(* Logix 5000 AddOnInstructionDefinition export Banner_K50ProTouch_PD_v4; software revision 33.00 *)

TYPE Banner_K50Pro_4State_v4 :   // Process Data for Four State Mode. This mode is only available in Touch models.
STRUCT
   Touch_Status : SINT;   // 0 = Inactive, 1 = Active. Only active for Touch models.
   In_State : SINT;   // Curent State. 0 = State 1, 1 = State 2, 2 = State 3, 3 = State 4
   Job_Control : SINT;   // 0 = Off, 1 = On
END_STRUCT
END_TYPE

TYPE Banner_K50Pro_MC_v4 :   // Process Data for Multicolor
STRUCT
   Touch_Status : SINT;   // 0 = Inactive, 1 = Active. Only active for Touch models.
   In_State : SINT;   // Curent State. 0 = State 1, 1 = State 2, 2 = State 3, 3 = State 4
   Out_State : SINT;   // Set Output State. 0 = State 1, 1 = State 2, 2 = State 3, 3 = State 4
END_STRUCT
END_TYPE

TYPE Banner_K50ProTouch_Adv_v4 :   // Advanced Process Data information for a Banner K50 Pro Touch.
STRUCT
   Touch_Status : SINT;   // 0 = Inactive, 1 = Active.
   Type : SINT;   // 0 = Off, 1 = Steady, 2 = Flash, 3 = Two Color Flash, 4 = 50/50, 5 = 50/50 Rotate, 6 = Chase, 7 = Intensity Sweep, 8 = Sequence.
   Direction : SINT;   // 0 = CCW, 1 = CW.
   Pattern : SINT;   // 0 = Flash, 1 = Strobe, 2 = Three Pulse, 3 = SOS, 4 = Random.
   Speed : SINT;   // 0 = Slow, 1 = Medium, 2 = Fast, 3 = Custom.
   Vibration_Feedback : SINT;   // 0 = Off, 1 = On, 2 = Animation Pattern. Not available in all models.
   Dynamic_Sequence : INT;   // 0 to 255. Value describing the LED position on the device.
   Sequence_Start_Location : SINT;   // 0 = LED 1, 1 = LED 2, 2 = LED 3, 3 = LED 4, 4 = LED 5, 5 = LED 6, 6 = LED 7, 7 = LED 8.
   Color_1 : SINT;   // 0 = Green, 1 = Red, 2 = Orange, 3 = Amber, 4 = Yellow, 5 = Lime Green, 6 = Spring Green, 7 = Cyan, 8 = Sky Blue, 9 = Blue, 10 = Violet, 11 = Magenta, 12 = Rose, 13 = White, 14 = Custom 1, 15 = Custom 2.
   Color_1_Intensity : SINT;   // 0 = High, 1 = Medium, 2 = Low, 3 = Off, 4 = Custom.
   Color_2 : SINT;   // 0 = Green, 1 = Red, 2 = Orange, 3 = Amber, 4 = Yellow, 5 = Lime Green, 6 = Spring Green, 7 = Cyan, 8 = Sky Blue, 9 = Blue, 10 = Violet, 11 = Magenta, 12 = Rose, 13 = White, 14 = Custom 1, 15 = Custom 2.
   Color_2_Intensity : SINT;   // 0 = High, 1 = Medium, 2 = Low, 3 = Off, 4 = Custom.
END_STRUCT
END_TYPE

TYPE Banner_K50ProTouch_LEDControl_v4 :   // LED Control Process Data for a K50 Pro Touch.
STRUCT
   Touch_Status : SINT;   // 0 = Inactive, 1 = Active.
   LED_1_Color : SINT;   // 0 = Green, 1 = Red, 2 = Orange, 3 = Amber, 4 = Yellow, 5 = Lime Green, 6 = Spring Green, 7 = Cyan, 8 = Sky Blue, 9 = Blue, 10 = Violet, 11 = Magenta, 12 = Rose, 13 = White, 14 = Custom 1, 15 = Custom 2.
   LED_1_Intensity : SINT;   // 0 to 10 (0 to 100%).
   LED_2_Color : SINT;   // 0 = Green, 1 = Red, 2 = Orange, 3 = Amber, 4 = Yellow, 5 = Lime Green, 6 = Spring Green, 7 = Cyan, 8 = Sky Blue, 9 = Blue, 10 = Violet, 11 = Magenta, 12 = Rose, 13 = White, 14 = Custom 1, 15 = Custom 2.
   LED_2_Intensity : SINT;   // 0 to 10 (0 to 100%).
   LED_3_Color : SINT;   // 0 = Green, 1 = Red, 2 = Orange, 3 = Amber, 4 = Yellow, 5 = Lime Green, 6 = Spring Green, 7 = Cyan, 8 = Sky Blue, 9 = Blue, 10 = Violet, 11 = Magenta, 12 = Rose, 13 = White, 14 = Custom 1, 15 = Custom 2.
   LED_3_Intensity : SINT;   // 0 to 10 (0 to 100%).
   LED_4_Color : SINT;   // 0 = Green, 1 = Red, 2 = Orange, 3 = Amber, 4 = Yellow, 5 = Lime Green, 6 = Spring Green, 7 = Cyan, 8 = Sky Blue, 9 = Blue, 10 = Violet, 11 = Magenta, 12 = Rose, 13 = White, 14 = Custom 1, 15 = Custom 2.
   LED_4_Intensity : SINT;   // 0 to 10 (0 to 100%).
   LED_5_Color : SINT;   // 0 = Green, 1 = Red, 2 = Orange, 3 = Amber, 4 = Yellow, 5 = Lime Green, 6 = Spring Green, 7 = Cyan, 8 = Sky Blue, 9 = Blue, 10 = Violet, 11 = Magenta, 12 = Rose, 13 = White, 14 = Custom 1, 15 = Custom 2.
   LED_5_Intensity : SINT;   // 0 to 10 (0 to 100%).
   LED_6_Color : SINT;   // 0 = Green, 1 = Red, 2 = Orange, 3 = Amber, 4 = Yellow, 5 = Lime Green, 6 = Spring Green, 7 = Cyan, 8 = Sky Blue, 9 = Blue, 10 = Violet, 11 = Magenta, 12 = Rose, 13 = White, 14 = Custom 1, 15 = Custom 2.
   LED_6_Intensity : SINT;   // 0 to 10 (0 to 100%).
   LED_7_Color : SINT;   // 0 = Green, 1 = Red, 2 = Orange, 3 = Amber, 4 = Yellow, 5 = Lime Green, 6 = Spring Green, 7 = Cyan, 8 = Sky Blue, 9 = Blue, 10 = Violet, 11 = Magenta, 12 = Rose, 13 = White, 14 = Custom 1, 15 = Custom 2.
   LED_7_Intensity : SINT;   // 0 to 10 (0 to 100%).
   LED_8_Color : SINT;   // 0 = Green, 1 = Red, 2 = Orange, 3 = Amber, 4 = Yellow, 5 = Lime Green, 6 = Spring Green, 7 = Cyan, 8 = Sky Blue, 9 = Blue, 10 = Violet, 11 = Magenta, 12 = Rose, 13 = White, 14 = Custom 1, 15 = Custom 2.
   LED_8_Intensity : SINT;   // 0 to 10 (0 to 100%).
   Vibration_Feedback : SINT;   // 0 = Off, 1 = On, 2 = Pattern.
   Vibration_Pattern : SINT;   // 0 = Off, 1 = On, 2 = 3 Pulses, 3 = SOS, 4 = Random.
   Vibration_Speed : SINT;   // 0 = Slow, 1 = Medium, 2 = Fast, 3 = Custom.
END_STRUCT
END_TYPE

TYPE Banner_K50ProTouch_PDIO_v4 :   // UDT that records the converted prcoess data.
STRUCT
   PD_MultiColor_State : Banner_K50Pro_MC_v4;   // Only active when Operation Mode set to 0. State tells the light which of the four states it should be in. 0 = State 1, 1 = State 2, 2 = State 3, 3 = State 4.
   PD_FourState_Job_Input : Banner_K50Pro_4State_v4;   // Only active when Operation Mode set to 1. Job Input tells the light how it should behave. 0 - Off, 1 = ON
   PD_Advanced : Banner_K50ProTouch_Adv_v4;   // Only active when Operation Mode set to 2.
   PD_LED : Banner_K50ProTouch_LEDControl_v4;   // Only active when Operation Mode set to 3.
   PDO_DT : SINT[10];
   PDI_DT : SINT[2];
END_STRUCT
END_TYPE

ADD_ON_INSTRUCTION Banner_K50ProTouch_PD_v4   (* revision 4.0, vendor Banner Engineering *)
// Takes the raw SINT information and converts that data into actual information.
VAR_IN_OUT
   Process_Data : Banner_K50ProTouch_PDIO_v4; {required}
END_VAR
VAR_INPUT
   Operation_Mode : SINT; {required}   // Linked from Parameters AOI or entered manually.
   Byte_Swap : BOOL; {required}
END_VAR
VAR
   PDO_Temp : SINT[10]; {access None}
   PDI_Temp : SINT[2]; {access None}
END_VAR

ROUTINE Logic   (* ladder *)
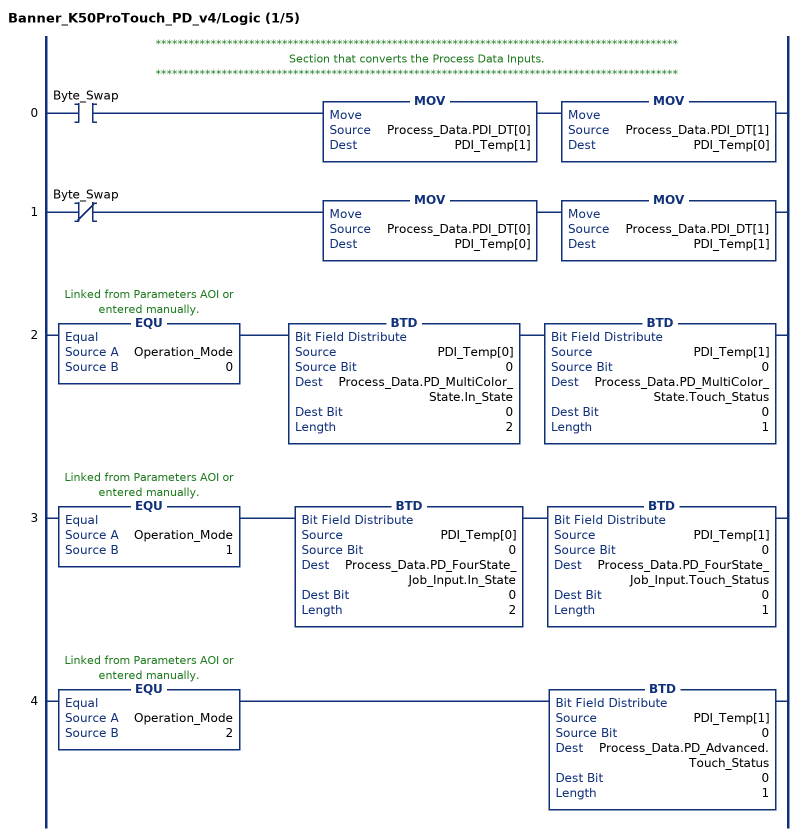
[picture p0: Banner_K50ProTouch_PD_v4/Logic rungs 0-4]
   // ***********************************************************************************************
   // Section that converts the Process Data Inputs.
   // ***********************************************************************************************
   0: XIC(Byte_Swap)MOV(Process_Data.PDI_DT[0],PDI_Temp[1])MOV(Process_Data.PDI_DT[1],PDI_Temp[0]);
   1: XIO(Byte_Swap)MOV(Process_Data.PDI_DT[0],PDI_Temp[0])MOV(Process_Data.PDI_DT[1],PDI_Temp[1]);
   2: EQU(Operation_Mode,0)BTD(PDI_Temp[0],0,Process_Data.PD_MultiColor_State.In_State,0,2)BTD(PDI_Temp[1],0,Process_Data.PD_MultiColor_State.Touch_Status,0,1);
   3: EQU(Operation_Mode,1)BTD(PDI_Temp[0],0,Process_Data.PD_FourState_Job_Input.In_State,0,2)BTD(PDI_Temp[1],0,Process_Data.PD_FourState_Job_Input.Touch_Status,0,1);
   4: EQU(Operation_Mode,2)BTD(PDI_Temp[1],0,Process_Data.PD_Advanced.Touch_Status,0,1);
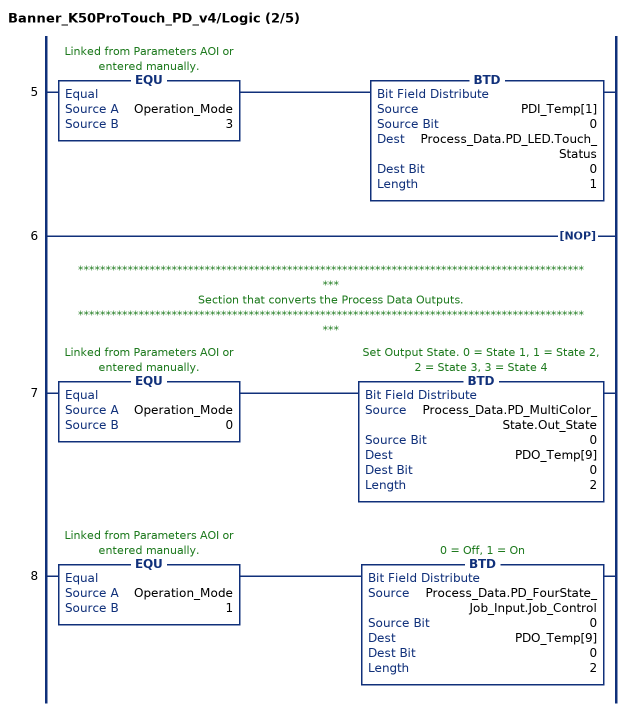
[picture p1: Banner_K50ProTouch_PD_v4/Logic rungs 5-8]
   5: EQU(Operation_Mode,3)BTD(PDI_Temp[1],0,Process_Data.PD_LED.Touch_Status,0,1);
   6: NOP();
   // ***********************************************************************************************
   // Section that converts the Process Data Outputs.
   // ***********************************************************************************************
   7: EQU(Operation_Mode,0)BTD(Process_Data.PD_MultiColor_State.Out_State,0,PDO_Temp[9],0,2);
   8: EQU(Operation_Mode,1)BTD(Process_Data.PD_FourState_Job_Input.Job_Control,0,PDO_Temp[9],0,2);
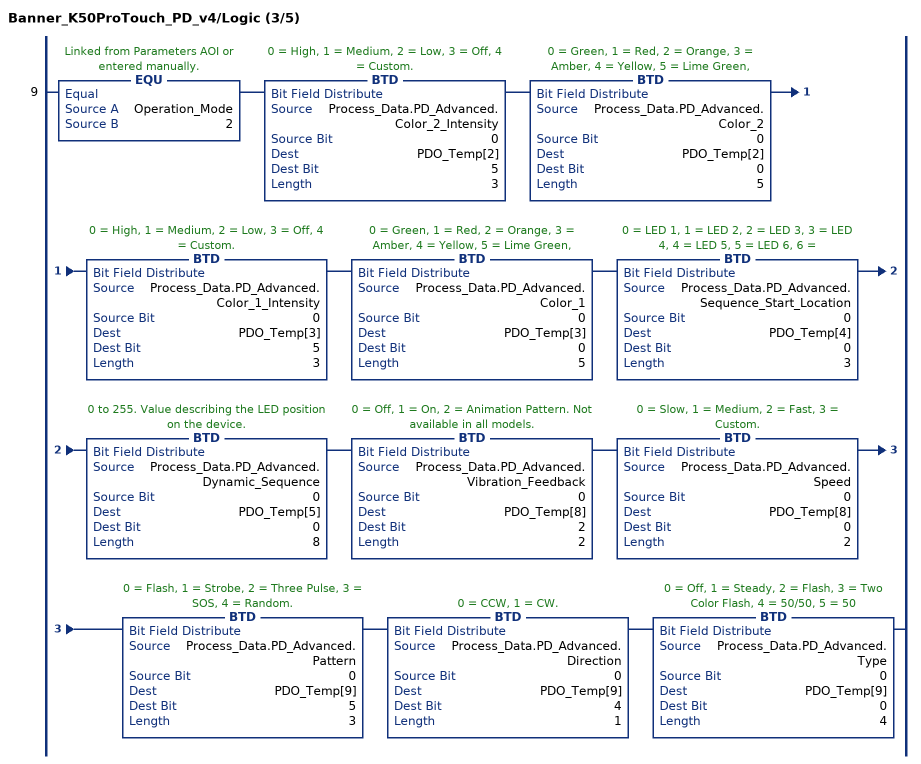
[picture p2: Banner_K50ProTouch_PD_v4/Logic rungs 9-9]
   9: EQU(Operation_Mode,2)BTD(Process_Data.PD_Advanced.Color_2_Intensity,0,PDO_Temp[2],5,3)BTD(Process_Data.PD_Advanced.Color_2,0,PDO_Temp[2],0,5)BTD(Process_Data.PD_Advanced.Color_1_Intensity,0,PDO_Temp[3],5,3)BTD(Process_Data.PD_Advanced.Color_1,0,PDO_Temp[3],0,5)BTD(Process_Data.PD_Advanced.Sequence_Start_Location,0,PDO_Temp[4],0,3)BTD(Process_Data.PD_Advanced.Dynamic_Sequence,0,PDO_Temp[5],0,8)BTD(Process_Data.PD_Advanced.Vibration_Feedback,0,PDO_Temp[8],2,2)BTD(Process_Data.PD_Advanced.Speed,0,PDO_Temp[8],0,2)BTD(Process_Data.PD_Advanced.Pattern,0,PDO_Temp[9],5,3)BTD(Process_Data.PD_Advanced.Direction,0,PDO_Temp[9],4,1)BTD(Process_Data.PD_Advanced.Type,0,PDO_Temp[9],0,4);
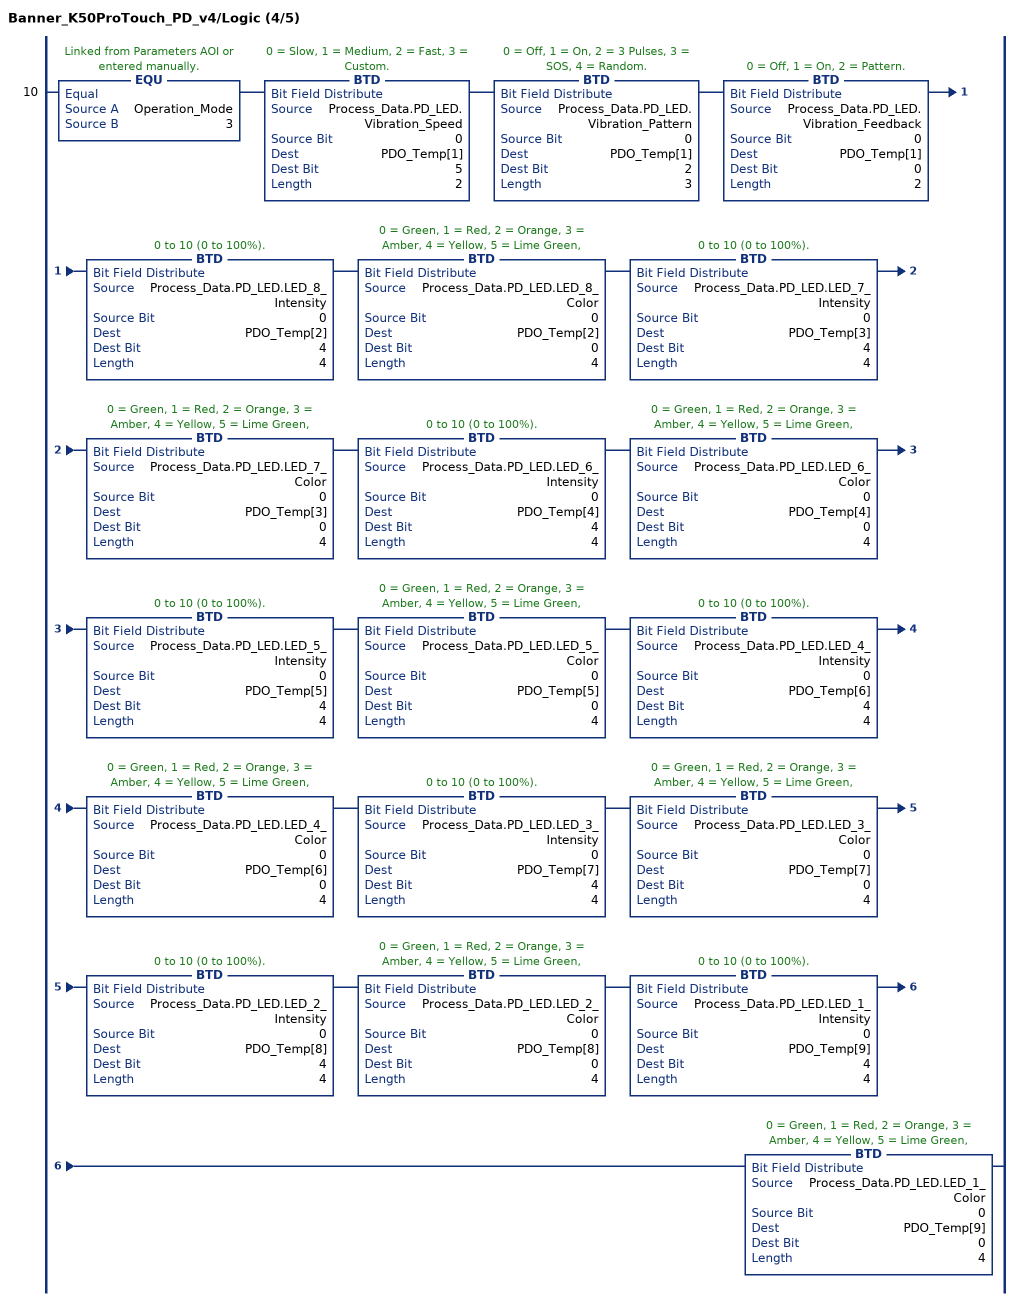
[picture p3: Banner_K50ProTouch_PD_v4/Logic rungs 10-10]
   10: EQU(Operation_Mode,3)BTD(Process_Data.PD_LED.Vibration_Speed,0,PDO_Temp[1],5,2)BTD(Process_Data.PD_LED.Vibration_Pattern,0,PDO_Temp[1],2,3)BTD(Process_Data.PD_LED.Vibration_Feedback,0,PDO_Temp[1],0,2)BTD(Process_Data.PD_LED.LED_8_Intensity,0,PDO_Temp[2],4,4)BTD(Process_Data.PD_LED.LED_8_Color,0,PDO_Temp[2],0,4)BTD(Process_Data.PD_LED.LED_7_Intensity,0,PDO_Temp[3],4,4)BTD(Process_Data.PD_LED.LED_7_Color,0,PDO_Temp[3],0,4)BTD(Process_Data.PD_LED.LED_6_Intensity,0,PDO_Temp[4],4,4)BTD(Process_Data.PD_LED.LED_6_Color,0,PDO_Temp[4],0,4)BTD(Process_Data.PD_LED.LED_5_Intensity,0,PDO_Temp[5],4,4)BTD(Process_Data.PD_LED.LED_5_Color,0,PDO_Temp[5],0,4)BTD(Process_Data.PD_LED.LED_4_Intensity,0,PDO_Temp[6],4,4)BTD(Process_Data.PD_LED.LED_4_Color,0,PDO_Temp[6],0,4)BTD(Process_Data.PD_LED.LED_3_Intensity,0,PDO_Temp[7],4,4)BTD(Process_Data.PD_LED.LED_3_Color,0,PDO_Temp[7],0,4)BTD(Process_Data.PD_LED.LED_2_Intensity,0,PDO_Temp[8],4,4)BTD(Process_Data.PD_LED.LED_2_Color,0,PDO_Temp[8],0,4)BTD(Process_Data.PD_LED.LED_1_Intensity,0,PDO_Temp[9],4,4)BTD(Process_Data.PD_LED.LED_1_Color,0,PDO_Temp[9],0,4);
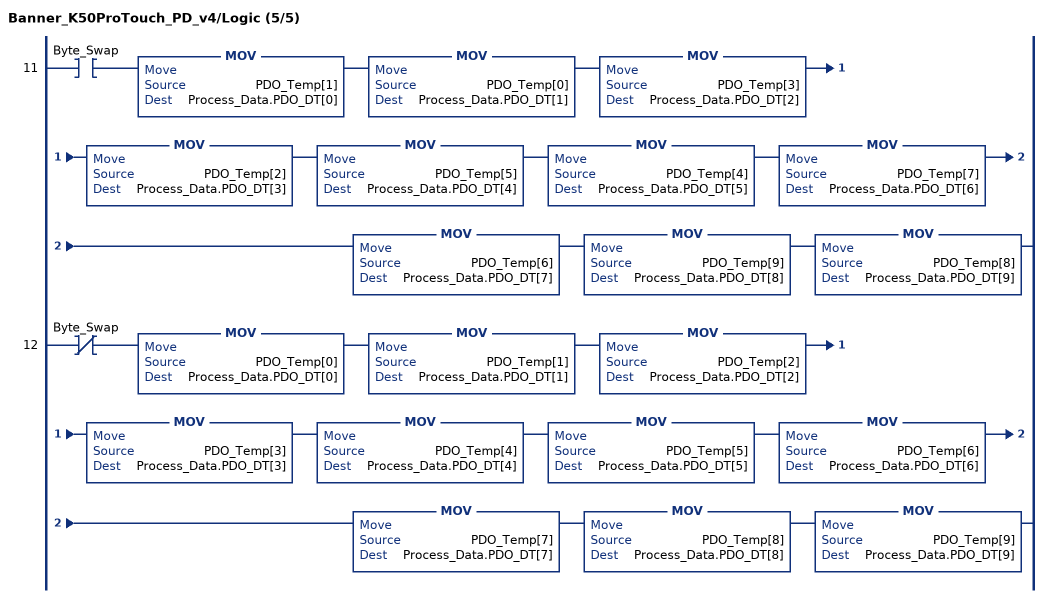
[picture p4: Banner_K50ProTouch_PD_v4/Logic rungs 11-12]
   11: XIC(Byte_Swap)MOV(PDO_Temp[1],Process_Data.PDO_DT[0])MOV(PDO_Temp[0],Process_Data.PDO_DT[1])MOV(PDO_Temp[3],Process_Data.PDO_DT[2])MOV(PDO_Temp[2],Process_Data.PDO_DT[3])MOV(PDO_Temp[5],Process_Data.PDO_DT[4])MOV(PDO_Temp[4],Process_Data.PDO_DT[5])MOV(PDO_Temp[7],Process_Data.PDO_DT[6])MOV(PDO_Temp[6],Process_Data.PDO_DT[7])MOV(PDO_Temp[9],Process_Data.PDO_DT[8])MOV(PDO_Temp[8],Process_Data.PDO_DT[9]);
   12: XIO(Byte_Swap)MOV(PDO_Temp[0],Process_Data.PDO_DT[0])MOV(PDO_Temp[1],Process_Data.PDO_DT[1])MOV(PDO_Temp[2],Process_Data.PDO_DT[2])MOV(PDO_Temp[3],Process_Data.PDO_DT[3])MOV(PDO_Temp[4],Process_Data.PDO_DT[4])MOV(PDO_Temp[5],Process_Data.PDO_DT[5])MOV(PDO_Temp[6],Process_Data.PDO_DT[6])MOV(PDO_Temp[7],Process_Data.PDO_DT[7])MOV(PDO_Temp[8],Process_Data.PDO_DT[8])MOV(PDO_Temp[9],Process_Data.PDO_DT[9]);
END_ROUTINE
END_ADD_ON_INSTRUCTION
